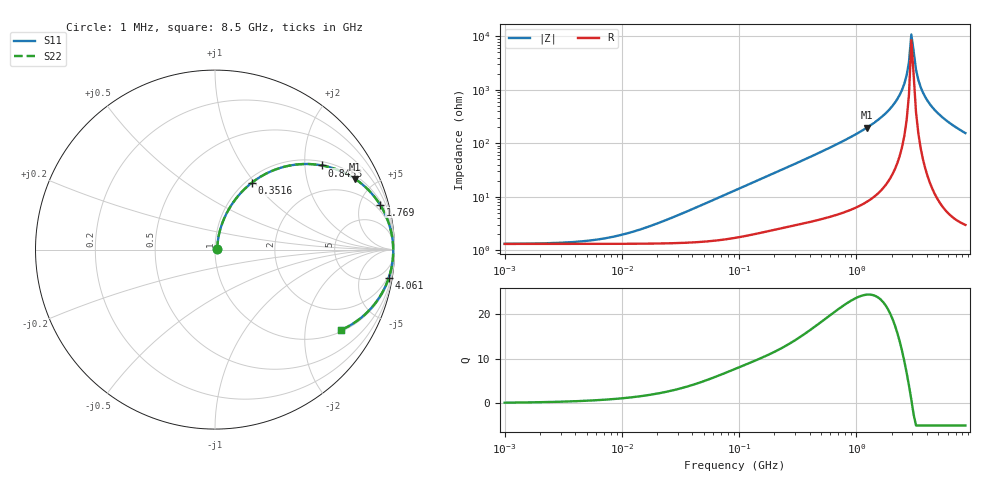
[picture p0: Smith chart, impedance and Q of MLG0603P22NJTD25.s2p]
! S-Parameter Data Generated by TDK Corporation
! Copyright(C) 2025 TDK Corporation.
! All Rights Reserved.
! TDK P/N: MLG0603P22NJTD25 (SMD / SMT Inductor (Coil))
! Property: L=22nH at 500MHz
! Size(LxWxT): 0.6x0.3x0.3mm
! Model Type: s2p (Touchstone File Format Version 1.0)
! Frequency: DC=Yes Start=1MHz Stop=8500MHz 198points Log-sweep
! Model Generated on Feb. 6, 2025
! Terms and conditions regarding TDK Simulation Models:
! 1)This simulation model is being provided solely for informational
!  purposes. Please refer to the specifications of the products in
!  terms of detailed characteristics of such products.
! 2)In no event shall TDK Corporation of any of its subsidiaries be
!  liable for any loss or damage arising, directly or indirectly,
!  from any information contained in this simulation model, including,
!  but not limited to loss or damages arising from any inaccuracies,
!  omissions or errors in connection with such information.
! 3)Any and all copyrights on this simulation model are owned by
!  TDK Corporation.  Duplication or redistribution of this simulation
!  model without prior written permission from TDK Corporation
!  is prohibited.
! 4)This simulation model is subject to any modification or change
!  without any prior notice.
! 5)Neither TDK Corporation nor any of its subsidiaries shall make any
!  warranty, express or implied, including but not limited to the
!  correctness, implied warranties of merchantability and fitness for
!  a particular purpose with respect to this simulation models.
! 6)The use of this simulation model shall be deemed to have consented
!  to the terms and conditions hereof.
! Port Assignments:
!  1 ---@@@--- 2
! Applicable Conditions:
!  Temperature = 25 degC
!  DC Bias Current = 0 A
!  Small Signal Operation
# Hz S MA R 50
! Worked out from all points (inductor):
!   197 points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, 1 MHz to 8.5 GHz, reference 50 ohm
!   read as one part in series: L = 22.7 nH near 29.07 MHz
!   highest Q = 24.4 at 1.223 GHz (marker M1), where L = 25.3 nH
!   self-resonance near 2.94 GHz
!   S11 on the Smith chart (normalised r, x): 1 MHz: 1.03, +0.00; 351.6 MHz: 1.06, +0.97; 845.3 MHz: 1.11, +2.45; 1.769 GHz: 1.33, +7.21; 4.061 GHz: 1, -12; 8.5 GHz: 1.06, -3.10
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1000000  0.01301 6.2  0.9871 -0.1  0.9871 -0.1  0.01301 6.2
4587603  0.01448 26.3  0.987 -0.4  0.987 -0.4  0.01448 26.3
9601846  0.01878 45.5  0.9869 -0.8  0.9869 -0.8  0.01878 45.5
2.10461e7  0.0325 64.4  0.9864 -1.7  0.9864 -1.7  0.0325 64.4
9.219544e7  0.1282 75.3  0.9753 -7.3  0.9753 -7.3  0.1282 75.3
2.020814e8  0.2646 69.8  0.9418 -15.3  0.9418 -15.3  0.2646 69.8
3.516439e8  0.4251 61.2  0.8779 -25.1  0.8779 -25.1  0.4251 61.2
4.229561e8  0.4912 57.2  0.8423 -29.4  0.8423 -29.4  0.4912 57.2
8.453103e8  0.7581 38.2  0.6194 -49.2  0.6194 -49.2  0.7581 38.2
1.222927e9  0.8752 26.7  0.4493 -61.0  0.4493 -61.0  0.8752 26.7
1.769233e9  0.9526 15.3  0.264 -72.1  0.264 -72.1  0.9526 15.3
1.940355e9  0.9654 12.5  0.2171 -74.6  0.2171 -74.6  0.9654 12.5
2.228565e9  0.98 8.4  0.1467 -78.0  0.1467 -78.0  0.98 8.4
2.559585e9  0.9891 4.4  0.07653 -79.6  0.07653 -79.6  0.9891 4.4
2.680511e9  0.9909 3.0  0.05322 -78.7  0.05322 -78.7  0.9909 3.0
2.80715e9  0.9922 1.7  0.03013 -74.1  0.03013 -74.1  0.9922 1.7
2.939772e9  0.9929 0.3  0.009143 -38.6  0.009143 -38.6  0.9929 0.3
3.224109e9  0.9925 -2.4  0.04181 78.4  0.04181 78.4  0.9925 -2.4
3.37643e9  0.9914 -3.7  0.06516 80.6  0.06516 80.6  0.9914 -3.7
4.061159e9  0.981 -9.2  0.1597 78.6  0.1597 78.6  0.981 -9.2
5.610304e9  0.9382 -19.1  0.3272 69.7  0.3272 69.7  0.9382 -19.1
8.5e9  0.833 -32.5  0.5376 56.4  0.5376 56.4  0.833 -32.5
